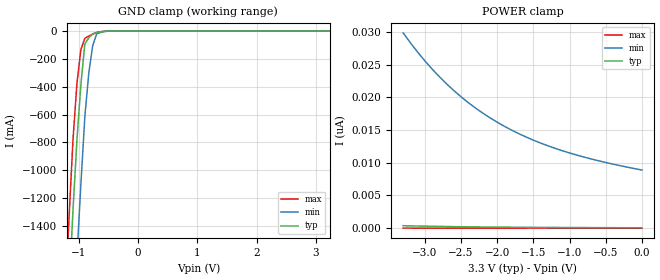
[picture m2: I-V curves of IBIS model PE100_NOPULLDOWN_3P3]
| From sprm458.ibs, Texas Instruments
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|   Model Cell PE100_NOPULLDOWN_3P3
|IDG09_PE100_NOPULLDOWN_3P3
[Model]   PE100_NOPULLDOWN_3P3
Model_type   Input
Polarity   Non-Inverting
Vinl =  0.8V
Vinh =  2V
C_comp   1.604p   1.5372p   1.8937p
[Model Spec]
Vinl   0.8V   0.8V   0.8V
Vinh   2V   2V   2V
[Temperature Range]   25   125   -40
[Voltage Range]   3.3   3   3.6
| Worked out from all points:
|   GND clamp passes 1 mA (typ) near -0.53 V on its own axis
[POWER_clamp]
|   voltage   I(typ)   I(min)   I(max)
-3.3V     375.2pA    29.86nA    7.807pA
-3.2V     350.3pA    28.34nA    7.212pA
-3V       305.8pA    25.58nA    5.764pA
-2.7V     250.4pA    22.07nA    4.547pA
-2.4V     206.4pA    19.2nA     3.642pA
-2.2V     182.4pA    17.6nA     3.118pA
-2V       161.4pA    16.2nA     2.602pA
-1.8V     143.8pA    14.99nA    2.176pA
-1.6V     128.7pA    13.94nA    1.856pA
-1.2V     104.7pA    12.21nA    1.368pA
-700mV    82.92pA    10.59nA    1.181pA
0V        62.12pA    8.892nA    692.8fA
[GND_clamp]
|   voltage   I(typ)   I(min)   I(max)
-3.3V     -22.54A    -23.36A    -22.09A
-1.233V   -2.454A    -3.359A    -1.924A
-1.167V   -1.863A    -2.762A    -1.341A
-1.1V     -1.287A    -2.174A    -780.3mA
-1.033V   -782.2mA   -1.619A    -375.5mA
-966.7mV  -384.2mA   -1.1A      -132.9mA
-900mV    -92.99mA   -616.1mA   -52.35mA
-833.3mV  -47.56mA   -302.3mA   -36.13mA
-766.7mV  -19.98mA   -103.7mA   -22.15mA
-700mV    -10.23mA   -20.38mA   -10.41mA
-500mV    -282.6uA   -891.2uA   -99.23uA
3.233V    60.56pA    9.405nA    581.8fA
